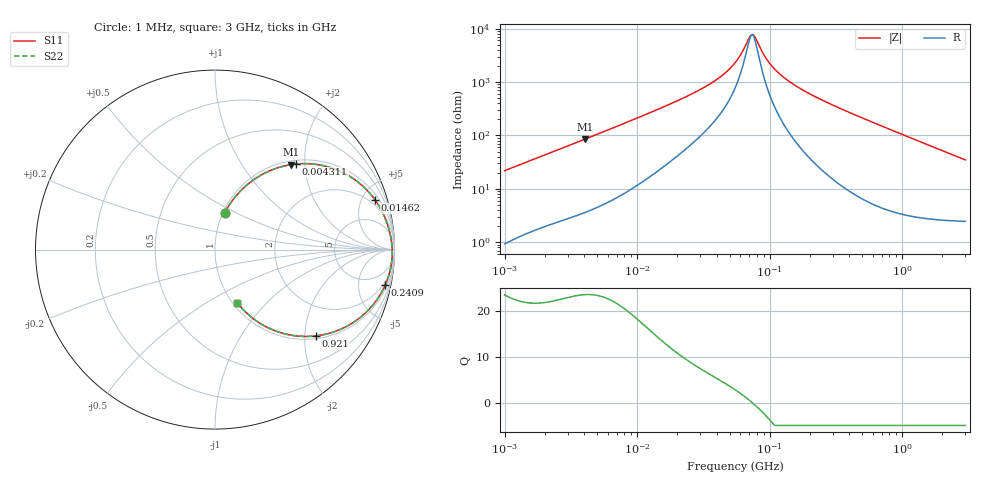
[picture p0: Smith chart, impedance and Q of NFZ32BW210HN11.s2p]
! NFZ32BW210HN11
# Hz S RI R 50
!Freq.(Hz) S11(Real) S11(Imag) S21(Real) S21(Imag) S12(Real) S12(Imag) S22(Real) S22(Imag)
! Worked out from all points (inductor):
!   401 points, 1 MHz to 3 GHz, reference 50 ohm
!   read as one part in series: L = 3.45 uH near 1.041 MHz
!   highest Q = 23.6 at 4.06 MHz (marker M1), where L = 3.34 uH
!   self-resonance near 72.49 MHz
!   S11 on the Smith chart (normalised r, x): 1 MHz: 1.02, +0.44; 4.311 MHz: 1.08, +1.81; 14.62 MHz: 1.45, +6.26; 240.9 MHz: 1.48, -9.53; 921 MHz: 1.07, -2.27; 3 GHz: 1.05, -0.69
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1000000  0.0536 0.205  0.9464 -0.205  0.9464 -0.205  0.0536 0.205
2014875  0.1673 0.3511  0.8327 -0.3511  0.8327 -0.3511  0.1673 0.3511
3823119  0.3973 0.4685  0.6027 -0.4685  0.6027 -0.4685  0.3973 0.4685
4059721  0.4249 0.4736  0.5751 -0.4736  0.5751 -0.4736  0.4249 0.4736
4310966  0.453 0.477  0.547 -0.477  0.547 -0.477  0.453 0.477
8345207  0.745 0.4117  0.255 -0.4117  0.255 -0.4117  0.745 0.4117
1.461624e7  0.8918 0.277  0.1082 -0.277  0.1082 -0.277  0.8918 0.277
3.456417e7  0.971 0.1064  0.029 -0.1064  0.029 -0.1064  0.971 0.1064
4.483659e7  0.9796 0.0677  0.0204 -0.0677  0.0204 -0.0677  0.9796 0.0677
5.477226e7  0.984 0.0399  0.016 -0.0399  0.016 -0.0399  0.984 0.0399
7.105049e7  0.9871 0.00497  0.0129 -0.00497  0.0129 -0.00497  0.9871 0.00497
7.544761e7  0.9874 -0.00312  0.0126 0.00312  0.0126 0.00312  0.9874 -0.00312
9.402997e7  0.9873 -0.0334  0.0127 0.0334  0.0127 0.0334  0.9873 -0.0334
1.103592e8  0.9857 -0.0565  0.0143 0.0565  0.0143 0.0565  0.9857 -0.0565
1.431579e8  0.9799 -0.0973  0.0201 0.0973  0.0201 0.0973  0.9799 -0.0973
2.094008e8  0.9607 -0.1671  0.0393 0.1671  0.0393 0.1671  0.9607 -0.1671
2.408952e8  0.9489 -0.1966  0.0511 0.1966  0.0511 0.1966  0.9489 -0.1966
4.480278e8  0.8429 -0.3485  0.1571 0.3485  0.1571 0.3485  0.8429 -0.3485
8.005644e8  0.628 -0.4687  0.372 0.4687  0.372 0.4687  0.628 -0.4687
9.209708e8  0.5616 -0.481  0.4384 0.481  0.4384 0.481  0.5616 -0.481
1.747494e9  0.2713 -0.4228  0.7287 0.4228  0.7287 0.4228  0.2713 -0.4228
3e9  0.1242 -0.2962  0.8758 0.2962  0.8758 0.2962  0.1242 -0.2962
